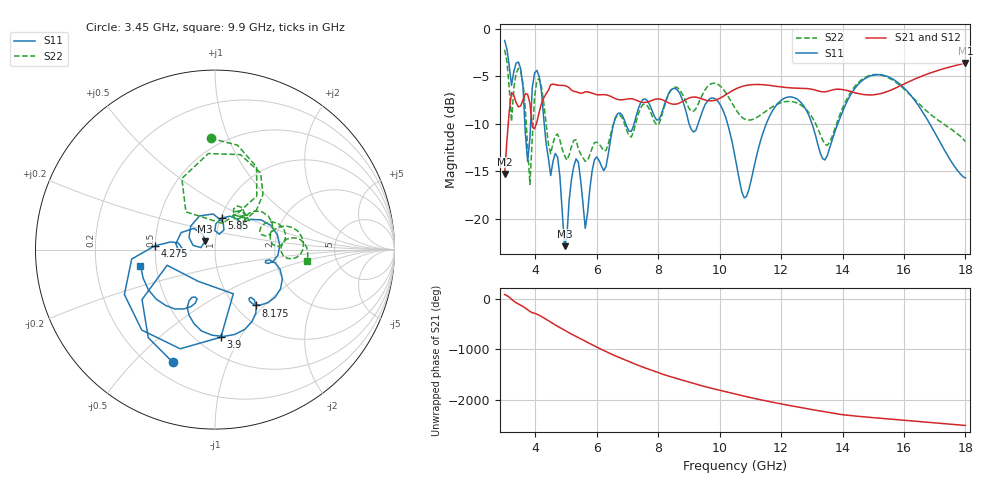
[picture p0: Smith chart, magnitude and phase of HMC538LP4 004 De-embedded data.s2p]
! Chelmsford, MA 01824
! http://www.hittite.com
! Tel: 978-250-3343
! Fax: 978-250-3373
! Device  :  HMC538LP4
! Description:  600 Analog Phase Shifter
! Frequency  :  6.0 GHz - 15.0 GHz
! Package  :  LP4  - 4x4 mm Quad Flatpack No-Lead (QFN) Plastic Package: 24 pin
! Ports  :  2 RF, 1 DC
!  Pin  3  = Rfin  = Port 1
!  Pin  16  = Rfout = Port 2
!  pin  21  = vCTL
! Voltages:  VCTL  = 0 to 5.0 Volts
! Currents :  Vb(V)  Vd(V)  Ib(mA)  Id(mA)
!  0.00  0.40  0.000000	0.480487
! Data:  The device was measured on evaluation board 111296-1.
!  Data was collected using a calibrated network analyzer.
!  The evaluation circuit board was modeled and simulated.This was use
!  to removed the evaluation board circuit from the measured data.
!  The reference plane is the center of the package pin.
! Misc:  Lot #
!Date Measured:  03 - 11 -2009
! Date:  03 - 17 -2009
! Note:
!  Hittite Microwave supplies this data as a sample of measured data at the
!  package pin for this package product.  Your particular data for this product
!  may vary.
!  Data was taken at 25 degrees C.
!  Hittite Microwave reserves the right to change this data at anytime.
# MHz S MA R 50
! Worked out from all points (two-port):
!   201 points, 3 GHz to 18 GHz, reference 50 ohm
!   highest |S21| = -3.57 dB at 18 GHz (marker M1); lowest = -15.3 dB at 3 GHz (marker M2)
!   |S21| within 3 dB of the highest: 10.38 GHz to 13.26 GHz (2.879 GHz wide, 24.4 % of centre); 15.47 GHz to end of sweep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
!   lowest |S11| = -22.9 dB at 4.95 GHz (marker M3), VSWR 1.15, Z = 44.6 + j4.13 ohm
!   |S11| at or under -10 dB: 4.29 GHz to 6.55 GHz (2.26 GHz wide, 41.7 % of centre); 10.26 GHz to 11.52 GHz (1.259 GHz wide, 11.6 % of centre); 16.84 GHz to end of sweep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
!   |S22| runs from -16.4 to -2.2 dB; largest |S21 - S12| = 0.0017
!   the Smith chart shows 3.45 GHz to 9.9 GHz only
!   S11 on the Smith chart (normalised r, x): 3.45 GHz: 0.29, -0.65; 3.9 GHz: 0.65, -0.83; 4.275 GHz: 0.50, +0.02; 5.85 GHz: 1.01, +0.37; 8.175 GHz: 1.23, -0.90; 9.9 GHz: 0.41, -0.09
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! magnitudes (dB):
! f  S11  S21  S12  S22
! 3 GHz  -1.2  -15.3  -15.3  -2.2
! 3.225 GHz  -5.9  -6.7  -6.7  -9.7
! 3.45 GHz  -3.5  -8.2  -8.2  -4.1
! 3.75 GHz  -14.0  -6.9  -6.9  -12.3
! 3.825 GHz  -11.5  -7.9  -7.9  -16.4
! 3.9 GHz  -6.2  -10.3  -10.3  -11.5
! 4.05 GHz  -4.3  -9.8  -9.8  -5.4
! 4.275 GHz  -9.5  -7.3  -7.3  -7.8
! 4.725 GHz  -13.5  -5.9  -5.9  -11.1
! 4.95 GHz  -22.9  -6.0  -6.0  -13.3
! 5.325 GHz  -13.7  -6.6  -6.6  -11.7
! 5.55 GHz  -18.4  -6.7  -6.7  -13.6
! 5.85 GHz  -14.9  -6.8  -6.8  -12.5
! 8.025 GHz  -9.6  -7.4  -7.4  -10.0
! 8.175 GHz  -8.2  -7.5  -7.5  -8.5
! 9.9 GHz  -7.4  -7.5  -7.5  -5.8
! 10.5 GHz  -13.5  -6.4  -6.4  -8.3
! 10.8 GHz  -17.8  -6.0  -6.0  -9.5
! 11.93 GHz  -7.7  -6.1  -6.1  -7.9
! 13.05 GHz  -10.4  -6.4  -6.4  -9.5
! 15.53 GHz  -5.1  -6.5  -6.5  -5.2
! 18 GHz  -15.7  -3.6  -3.6  -11.9
